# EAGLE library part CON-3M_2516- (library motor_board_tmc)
3M (TM) Pak 100 4-Wall Header Source: 3M
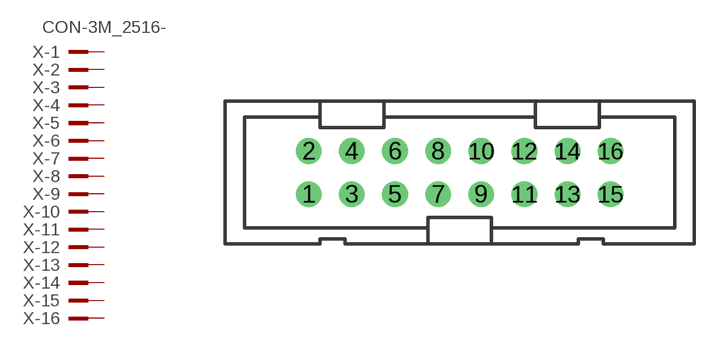
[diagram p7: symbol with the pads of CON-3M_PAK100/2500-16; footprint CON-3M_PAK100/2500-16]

Designator prefix X; gates -1=CON-3M_PINV -2=CON-3M_PIN -3=CON-3M_PIN -4=CON-3M_PIN -5=CON-3M_PIN -6=CON-3M_PIN -7=CON-3M_PIN -8=CON-3M_PIN -9=CON-3M_PIN -10=CON-3M_PIN -11=CON-3M_PIN -12=CON-3M_PIN -13=CON-3M_PIN -14=CON-3M_PIN -15=CON-3M_PIN -16=CON-3M_PIN

## CON-3M_2516- (MPN: D2516-5002-AR; OC_FARNELL: 9838376; OC_NEWARK: 12P7055)  [CON-3M_PAK100/2500-16]
1  -1:KL  pas
2  -2:KL  pas
3  -3:KL  pas
4  -4:KL  pas
5  -5:KL  pas
6  -6:KL  pas
7  -7:KL  pas
8  -8:KL  pas
9  -9:KL  pas
10  -10:KL  pas
11  -11:KL  pas
12  -12:KL  pas
13  -13:KL  pas
14  -14:KL  pas
15  -15:KL  pas
16  -16:KL  pas

## Footprint CON-3M_PAK100/2500-16 (pad centres in mm)
3M (TM) Pak 100 4-Wall Header Straight Source: 3M
drill 1 pad 1.422: 1 -8.89,-1.27; 2 -8.89,1.27; 3 -6.35,-1.27; 4 -6.35,1.27; 5 -3.81,-1.27; 6 -3.81,1.27; 7 -1.27,-1.27; 8 -1.27,1.27; 9 1.27,-1.27; 10 1.27,1.27; 11 3.81,-1.27; 12 3.81,1.27; 13 6.35,-1.27; 14 6.35,1.27; 15 8.89,-1.27; 16 8.89,1.27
